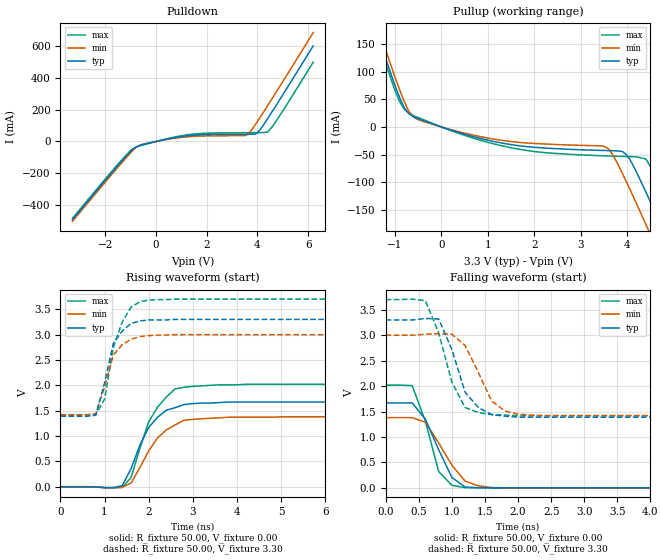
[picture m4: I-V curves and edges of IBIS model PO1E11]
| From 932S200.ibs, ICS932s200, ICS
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|   Model PO1E11
[Model]   PO1E11
Model_type   Output
Polarity   Non-Inverting
Vmeas =   1.50V
Cref =  20.00pF
Rref =  0.000
Vref =   1.50V
C_comp   5.50pF   5.00pF   6.00pF
[Temperature Range]   27.00   70.00   0.00
[Voltage Range]   3.30V   3.00V   3.70V
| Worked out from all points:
|   slope of the pulldown table from 0 to 0.495 V, typ, clamps not added: 28.9 ohm
|   slope of the pullup table from 0 to 0.495 V, typ, clamps not added: 37.7 ohm
|   rising waveform, R_fixture 50.00, V_fixture 0.00: 20-80 % time 579ps typ, 646ps min, 568ps max; typ from 0 V to 1.67 V
|   rising waveform, R_fixture 50.00, V_fixture 3.30: 20-80 % time 360ps typ, 372ps min, 369ps max; typ from 1.39 V to 3.3 V
|   falling waveform, R_fixture 50.00, V_fixture 0.00: 20-80 % time 348ps typ, 417ps min, 271ps max; typ from 1.67 V to 0 V
|   falling waveform, R_fixture 50.00, V_fixture 3.30: 20-80 % time 338ps typ, 347ps min, 343ps max; typ from 3.3 V to 1.39 V
[Pulldown]
| voltage   I(typ)   I(min)   I(max)
-3.3V     -490.2mA   -501.8mA   -482.9mA
-1.5V     -148.6mA   -160.5mA   -141.3mA
-1V       -59.86mA   -70.16mA   -55.59mA
-700mV    -28.18mA   -27.69mA   -30.26mA
300mV     10.71mA    9mA        12.18mA
1.3V      36.89mA    30.2mA     43.26mA
3.6V      45.65mA    42.52mA    55.18mA
3.9V      46.6mA     102mA      55.47mA
4V        54.75mA    125.7mA    55.57mA
4.4V      142.8mA    224.3mA    59.01mA
4.8V      242.4mA    325.4mA    142.6mA
6.2V      601mA      684.6mA    498.1mA
[Pullup]
| voltage   I(typ)   I(min)   I(max)
-3.3V     655.7mA    671.1mA    646.1mA
-1.5V     196.6mA    212.6mA    186.7mA
-900mV    53.14mA    67.41mA    45.92mA
-600mV    18.38mA    17.65mA    20.45mA
1.4V      -30.61mA   -25.38mA   -35.92mA
3.5V      -42.6mA    -34.96mA   -52.28mA
3.7V      -43.04mA   -51.97mA   -52.84mA
4V        -51.32mA   -102.4mA   -53.55mA
4.4V      -117.3mA   -176.1mA   -57.95mA
4.8V      -191.7mA   -251.5mA   -120.6mA
5.2V      -267.5mA   -327.7mA   -195mA
6.2V      -459.4mA   -519.6mA   -386.1mA
[Ramp]
| variable   typ   min   max
dV/dt_r   1.00/574.31p   825.60m/629.58p   1.21/565.64p
dV/dt_f   1.15/300.00p   947.40m/300.00p   1.37/300.00p
[Rising Waveform]
R_fixture = 50.00
V_fixture = 0.00
V_fixture_min = 0.00
V_fixture_max = 0.00
| time   V(typ)   V(min)   V(max)
0s        0V         0V         0V
1.4ns     20.82mV    -9.41mV    -14.52mV
1.6ns     356.6mV    71.5mV     178.8mV
1.8ns     819.5mV    378.4mV    757.1mV
2ns       1.17V      706mV      1.28V
2.2ns     1.37V      965.5mV    1.57V
2.6ns     1.56V      1.22V      1.93V
2.8ns     1.62V      1.31V      1.96V
3.8ns     1.67V      1.37V      2.01V
10ns      1.67V      1.38V      2.02V
[Rising Waveform]
R_fixture = 50.00
V_fixture = 3.30
V_fixture_min = 3.00
V_fixture_max = 3.70
| time   V(typ)   V(min)   V(max)
0s        1.39V      1.42V      1.42V
800ps     1.41V      1.44V      1.42V
1ns       2.05V      1.97V      1.73V
1.2ns     2.83V      2.6V       2.75V
1.4ns     3.07V      2.8V       3.25V
1.6ns     3.22V      2.91V      3.54V
1.8ns     3.27V      2.96V      3.65V
2ns       3.29V      2.98V      3.68V
2.6ns     3.3V       3V         3.7V
10ns      3.3V       3V         3.7V
[Falling Waveform]
R_fixture = 50.00
V_fixture = 0.00
V_fixture_min = 0.00
V_fixture_max = 0.00
| time   V(typ)   V(min)   V(max)
0s        1.67V      1.38V      2.02V
400ps     1.67V      1.38V      2.01V
600ps     1.35V      1.29V      1.31V
800ps     751.8mV    885.4mV    323.2mV
1ns       205.8mV    446mV      50.44mV
1.2ns     15.26mV    132.6mV    3.53mV
1.4ns     4.24mV     39.86mV    1.26mV
1.6ns     1.08mV     7.07mV     398.1uV
1.8ns     348.3uV    1.88mV     142.1uV
10ns      0V         0V         -569nV
[Falling Waveform]
R_fixture = 50.00
V_fixture = 3.30
V_fixture_min = 3.00
V_fixture_max = 3.70
| time   V(typ)   V(min)   V(max)
0s        3.3V       3V         3.7V
600ps     3.33V      3.02V      3.68V
800ps     3.32V      3.03V      3.05V
1ns       2.72V      3.02V      2.08V
1.2ns     1.88V      2.8V       1.58V
1.4ns     1.58V      2.27V      1.48V
1.6ns     1.44V      1.71V      1.44V
1.8ns     1.41V      1.51V      1.43V
2.2ns     1.39V      1.43V      1.42V
10ns      1.39V      1.42V      1.42V
